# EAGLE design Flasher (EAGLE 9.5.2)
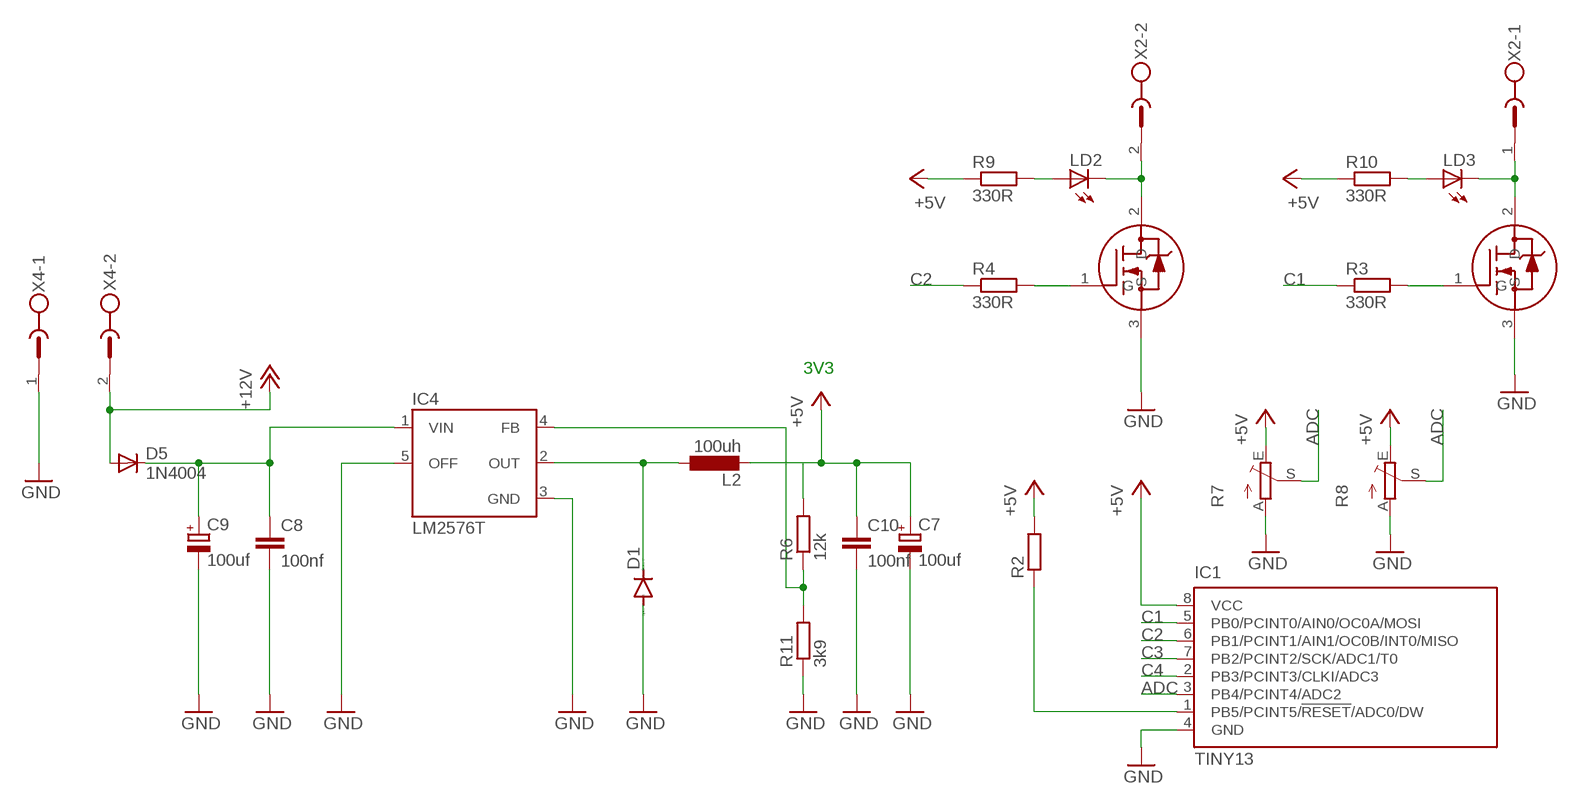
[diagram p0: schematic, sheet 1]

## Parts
C7  100uf  CPOL-EUE2.5-6  [E2,5-6]
C8  100nf  C-EUC0805K  [C0805K]
C9  100uf  CPOL-EUE2,5-6E  [E2,5-6E]
C10  100nf  C-EUC0805K  [C0805K]
D1  DIODE-DO214AA  [DO214AA]
D5  1N4004  [DO41-10]
IC1  TINY13  TINY13-20PU  [DIL08]
IC4  LM2576T  [TO220-5]
L2  100uh  L-EU6000-XXX-RC  [6000-XXXX-RC]
LD2  LED3MM  [LED3MM]
LD3  LED3MM  [LED3MM]
R2  R-EU_M0805  [M0805]
R3  330R  R-EU_M0805  [M0805]
R4  330R  R-EU_M0805  [M0805]
R6  12k  R-EU_M0805  [M0805]
R7  TRIM_EU-B25U  [B25U]
R8  TRIM_EU-B25P  [B25P]
R9  330R  R-EU_0204/2V  [0204V]
R10  330R  R-EU_0204/2V  [0204V]
R11  3k9  R-EU_M0805  [M0805]
U$1  20N03  [DPAK]
U$3  20N03  [DPAK]
X2  MSTBV2  [MSTBV2]
X4  MSTBV2  [MSTBV2]

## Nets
+5V: C7.+ C10.1 IC1.8(VCC) L2.2 R2.2 R6.2 R7.E R8.E R9.1 R10.1
+12V: D5.A X4.2
ADC: IC1.3(PB4/PCINT4/ADC2) R7.S R8.S
C1: IC1.5(PB0/PCINT0/AIN0/OC0A/MOSI) R3.1
C2: IC1.6(PB1/PCINT1/AIN1/OC0B/INT0/MISO) R4.1
C3: IC1.7(PB2/PCINT2/SCK/ADC1/T0)
C4: IC1.2(PB3/PCINT3/CLKI/ADC3)
GND: C7.- C8.2 C9.- C10.2 D1.A IC1.4(GND) IC4.3(GND) IC4.5(OFF) R7.A R8.A R11.1 U$1.3(S) U$3.3(S) X4.1
N$1: LD2.K(C) U$1.2(D) X2.2
N$4: R4.2 U$1.1(G)
N$5: IC1.1(PB5/PCINT5/!RESET!/ADC0/DW) R2.1
N$6: LD3.K(C) U$3.2(D) X2.1
N$7: R3.2 U$3.1(G)
N$11: D1.C IC4.2(OUT) L2.1
N$12: IC4.4(FB) R6.1 R11.2
N$13: LD2.A R9.2
N$14: LD3.A R10.2
N$15: C8.1 C9.+ D5.C IC4.1(VIN)

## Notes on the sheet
- 3V3

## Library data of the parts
C7 C9 = rcl:CPOL-EU: POLARIZED CAPACITOR, European symbol
C8 C10 = rcl:C-EU: CAPACITOR, European symbol
D1 = diode:DIODE-: DIODE
D5 = diode:1N4004: DIODE
IC1 = atmel:TINY13: 8-bit AVR Microcontroller with 1K Bytes In-System Programmable Flash Source: http://www.atmel.com/dyn/resources/prod_documents/2535S.pdf; MPN: ATTINY13-20PU; OC_FARNELL: 9171550; OC_NEWARK: 96K6521
IC4 = v-reg-3:LM2576: National Semiconductor 3.0A "Simple Switcher"(c) 52kHz, Vout 1.23-37V (HV: 57V), Vin 40V (HV: 60V), 50µA standby current
L2 = rcl:L-EU: INDUCTOR, European symbol
LD2 LD3 = led:LED: LED
R2-R4 R6 R9-R11 = rcl:R-EU_: RESISTOR, European symbol
R7 R8 = pot:TRIM_EU-: POTENTIOMETER
U$1 U$3 = 20n03:20N03
X2 X4 = con-phoenix-500:MSTBV2: PHOENIX; OC_FARNELL: unknown; OC_NEWARK: unknown

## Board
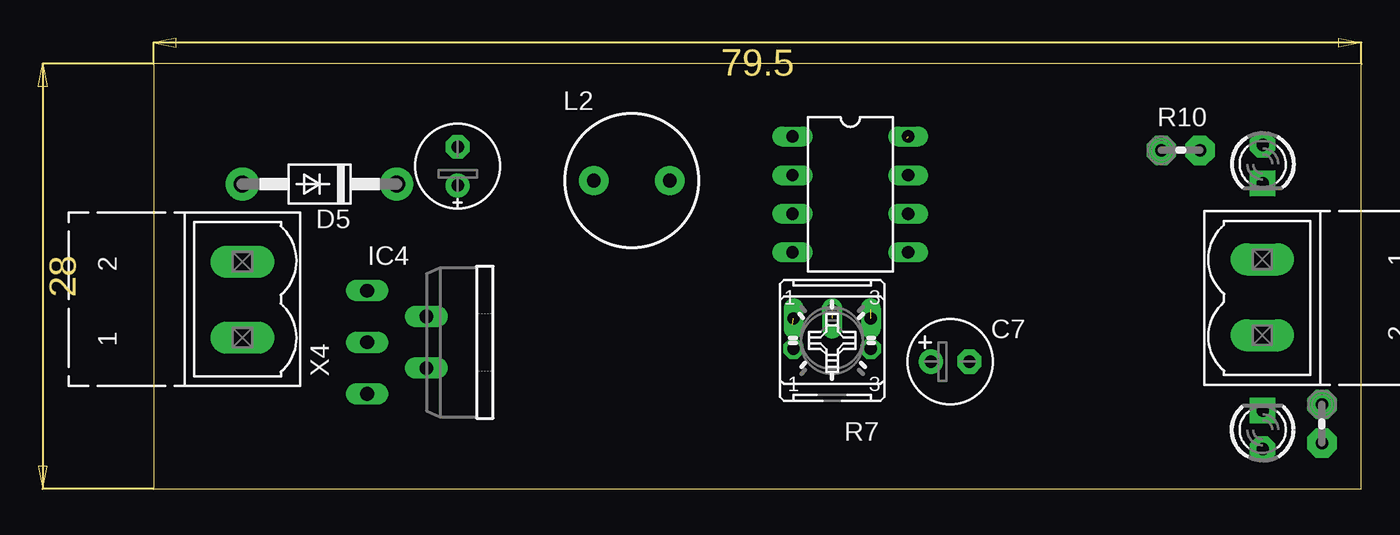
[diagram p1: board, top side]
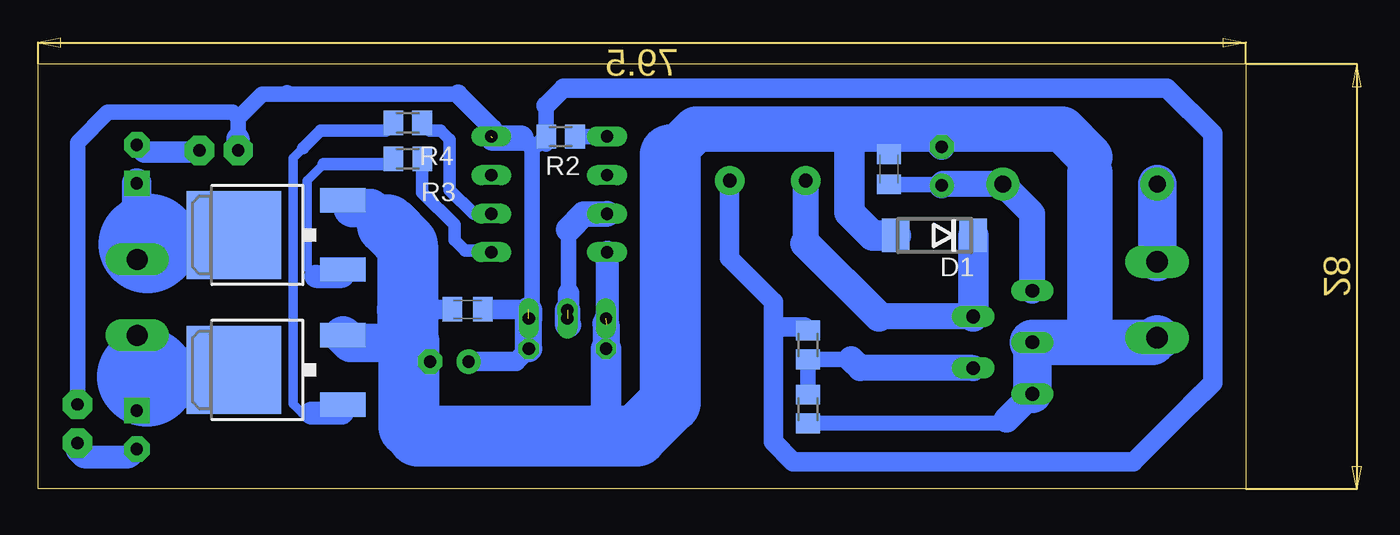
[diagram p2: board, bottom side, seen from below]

Size 87.1 x 29.7 mm. Coordinates in mm from the lower left corner, seen from the top.
Outline: 7.6,0 87.1,0 87.1,28 7.6,28 7.6,0
Copper layers (1*16): Top 0.035mm / dielectric 1.5mm / Bottom 0.035mm
Design rules "default": minimum track width 10mil, minimum drill 24mil, track to track 8mil, track to pad 8mil, pad to pad 8mil, via to via 8mil, smd to smd 8mil, copper to edge 40mil, drill to drill 8mil, minimum pad ring 10mil, minimum via ring 8mil, stop-mask expansion 4mil, vias tented up to drill 0mil, thermal gap 10mil

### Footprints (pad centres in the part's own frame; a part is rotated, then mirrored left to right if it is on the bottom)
E2,5-6 = drill 0.813 pad 1.6: + -1.27,0 | drill 0.813 pad 1.6 octagon: - 1.27,0
C0805K = smd 1.3 x 1.6: 1 -1,0; 2 1,0
E2,5-6E = drill 0.813 pad 1.575: + -1.27,0 | drill 0.813 pad 1.575 octagon: - 1.27,0
DO214AA = smd 1.8 x 2.2: A 2.55,0; C -2.55,0
DO41-10 = drill 1.118 pad 2.184: A 5.08,0; C -5.08,0
DIL08 = drill 0.813 long: 1 -3.81,-3.81; 2 -1.27,-3.81; 3 1.27,-3.81; 4 3.81,-3.81; 5 3.81,3.81; 6 1.27,3.81; 7 -1.27,3.81; 8 -3.81,3.81
TO220-5 = drill 0.9 long: 1 -3.4,-8.4; 2 -1.7,-4.5; 3 0,-8.4; 4 1.7,-4.5; 5 3.4,-8.4
6000-XXXX-RC = drill 0.9 pad 1.93: 1 -2.5,0; 2 2.5,0
LED3MM = drill 0.813 pad 1.676 octagon: A -1.27,0 | drill 0.813 pad 1.676 square: K 1.27,0
M0805 = smd 1.3 x 1.6: 1 -0.95,0; 2 0.95,0
B25U = drill 0.813 long: A 2.54,-0.889; E -2.54,-0.889; S 0,-0.889
B25P = drill 0.813 octagon: A -2.54,0; E 2.54,0; S 0,2.54
0204V = drill 0.813 pad 1.93 octagon: 1 -1.27,0; 2 1.27,0
DPAK = smd 1.6 x 3: 1 -2.28,-4.8; 3 2.28,-4.8 | smd 5.8 x 6.2: 2 0,2.38
MSTBV2 = drill 1.397 long: 1 -2.5,0; 2 2.5,0

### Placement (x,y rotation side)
C7  60.03,8.39 0 top
C8  31.1,21.06 90 bottom
C9  27.62,21.26 90 top
C10  58.83,11.83 180 bottom
D1  28.1,16.7 180 bottom
D5  18.53,20.08 180 top
IC1  53.46,19.4 270 top
IC4  30.06,9.66 270 top
L2  39.08,20.31 0 top
LD2  80.6,3.9 90 top
LD3  80.6,21.4 270 top
R2  52.7,23.2 180 bottom
R3  62.76,21.73 180 bottom
R4  62.77,24.11 180 bottom
R6  36.43,9.49 90 bottom
R7  52.26,10.34 180 top
R8  52.26,9.23 0 top
R9  84.5,4.3 270 top
R10  75.2,22.3 0 top
R11  36.43,5.27 90 bottom
U$1  71.83,7.84 90 bottom
U$3  71.83,16.73 90 bottom
X2  80.57,12.62 270 top
X4  13.45,12.46 90 top

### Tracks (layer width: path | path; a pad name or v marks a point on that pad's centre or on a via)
+5V  (2 unrouted)
  Bottom 1.016: R9.1 84.5,22.8 82.5,24.8 74.3,24.8 73.93,24.43 | 54.6,22.4 54.6,12 54.8,11.8 | 55.3,23.1 54.6,22.4 | R2.2 54.15,22.7 54.3,22.7 54.6,22.4 | R2.2 53.65,22.7 | 73.93,24.43 73.93,23.1 | 53.65,25.25 R2.2 | 73.93,24.43 72.36,26 70.8,26 | 70.8,26 59.45,26 | 36.66,10.67 R6.2 | 70.7,26.1 70.8,26 | 11.22,5.58 11.22,5.6
  Bottom 1.27: 57.18,23.3 57.18,23.73 59.45,26 | 38.7,10.67 36.66,10.67 | 38.7,10.67 38.7,3.1 37.4,1.8 15,1.8 11.22,5.58 9.8,7 9.8,23.4 12.8,26.4 52.5,26.4 53.65,25.25 | L2.2 41.58,15.21 38.7,12.33 38.7,10.67 | 54.83,11.83 54.8,11.8 | C7.+ 55.64,8.39 R8.E | C10.1 54.87,11.83 54.8,11.76
  Bottom 1.5: 73.93,23.1 R10.1
  Bottom 1.676: 57.18,23.1 55.3,23.1 | 57.18,23.3 IC1.8 57.27,23.24
  Bottom 1.778: R8.E R7.E 54.8,11.76
+12V
  Bottom 2.54: X4.2 D5.A
ADC  (1 unrouted)
  Bottom 1.016: 52.2,17.1 52.2,12.9
  Bottom 1.422: 52.2,12.9 52.2,10.79
  Bottom 1.676: 52.2,17.1 51.2,18.1 49.65,18.1 IC1.3 | 52.2,10.79 52.26,10.85 R8.S
C1
  Bottom 0.813: IC1.5 57.37,15.69 58.99,15.69 59.7,16.4 59.7,17.42 61.81,19.53 R3.1
C2
  Bottom 0.813: IC1.6 58.43,18.13 60,19.7 60,23 60.61,23.61 61.32,23.61 R4.1
GND  (1 unrouted)
  Bottom 0.813: U$3.3 66.53,18.51 66.4,18.51
  Bottom 1: 23.34,4.58 23.6,4.32 R11.1
  Bottom 1.016: C8.2 31.27,22.23 31.27,22.64 | X4.1 12.86,9.96
  Bottom 1.27: C9.- 27.62,23.52 27.8,23.7 | C8.2 31.1,23.7 | 49.72,3.62 49.6,3.5 | C10.2 62.75,11.83 62.78,11.8 | C7.- 62.61,9.7 62.7,9.7
  Bottom 1.422: 49.72,10.87 49.65,10.8
  Bottom 1.5: IC1.4 49.65,11.3 R7.A
  Bottom 1.676: 57.96,3.96 57.5,3.5
  Bottom 1.7: IC4.5 23.34,4.58 | 27.73,22.64 C9.-
  Bottom 1.778: 49.72,10.87 R8.A
  Bottom 2: R8.A 49.72,3.62 | D1.A 32.2,16.7 33.7,18.2 33.7,23.7
  Bottom 2.5: 17.87,21.87 17.87,20.84
  Bottom 2.54: U$1.3 66.53,9.62 62.78,9.62 | 64.1,17.4 65.21,18.51 66.4,18.51 | IC4.5 IC4.3
  Bottom 3: 17.87,9.66 13.75,9.66 X4.1 | IC4.3 17.87,9.66 | 17.87,21.87 19.7,23.7 27.8,23.7 31.1,23.7 | 31.2,23.7 33.7,23.7 43.79,23.7 45.5,21.99 | 17.87,20.84 17.87,9.66
  Bottom 3.81: 62.78,9.62 62.7,9.7 | 62.7,4.1 62.1,3.5
  Bottom 4: 62.7,9.7 62.7,4.1 62.2,4.1 | 62.1,3.5 57.5,3.5 49.6,3.5 47.7,3.5 45.5,5.7 45.5,21.99 | 62.78,9.62 62.78,11.8 62.78,16.08 64.1,17.4
N$1
  Bottom 1.93: 80,7.4 80,9.05 80.57,9.62 X2.2 | LD2.K 80.6,6.68 79.94,7.34
  Bottom 4: 79.94,7.34 74.71,7.34 U$1.2
  Bottom 6.452: 80,7.4 79.94,7.34
N$4
  Bottom 0.61: 69.4,22.7 69.65,22.45 70.3,21.8 70.3,5.6 69.7,5 69.1,5
  Bottom 0.813: R4.2 64.22,23.61 68.49,23.61 69.65,22.45
  Bottom 1.5: 69.1,5 67.09,5 67.03,5.06 U$1.1
N$5
  Bottom 1.016: R2.1 IC1.1
N$6
  Bottom 1.778: 79.9,16.1 79.9,15.8 79.9,15.29 80.07,15.12 X2.1
  Bottom 1.93: LD3.K 80.6,16.5 79.9,15.8
  Bottom 4: 79.77,16.23 74.71,16.23 U$3.2
  Bottom 6.452: 79.9,16.1 79.77,16.23
N$7
  Bottom 0.61: 68.3,21.4 69.4,20.3 69.4,14.6 68.8,14
  Bottom 0.813: 68.3,21.4 63.88,21.4 63.71,21.57 R3.2
  Bottom 1.5: 68.8,14 67.08,14 67.03,14.05 U$3.1
N$11
  Bottom 1.7: IC4.2 31.76,11.36 | L2.1 36.58,16.18
  Bottom 2: 31.76,11.36 36.58,16.18 | D1.C IC4.2
N$12
  Bottom 1.016: 33.57,8.54 R6.1 R11.2
  Bottom 1.7: IC4.4 32.99,7.96 33.57,8.54
N$13
  Bottom 1.5: R9.2 84.5,2.53 84.1,2.13 81.1,2.13 LD2.A
N$14
  Bottom 1.422: LD3.A 80.1,22.17 76.84,22.17 76.71,22.3 R10.2
N$15
  Bottom 1.016: C8.1 27.55,20.06 27.53,20.08
  Bottom 1.7: IC4.1 21.66,18.13 D5.C 27.53,20.08 C9.+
